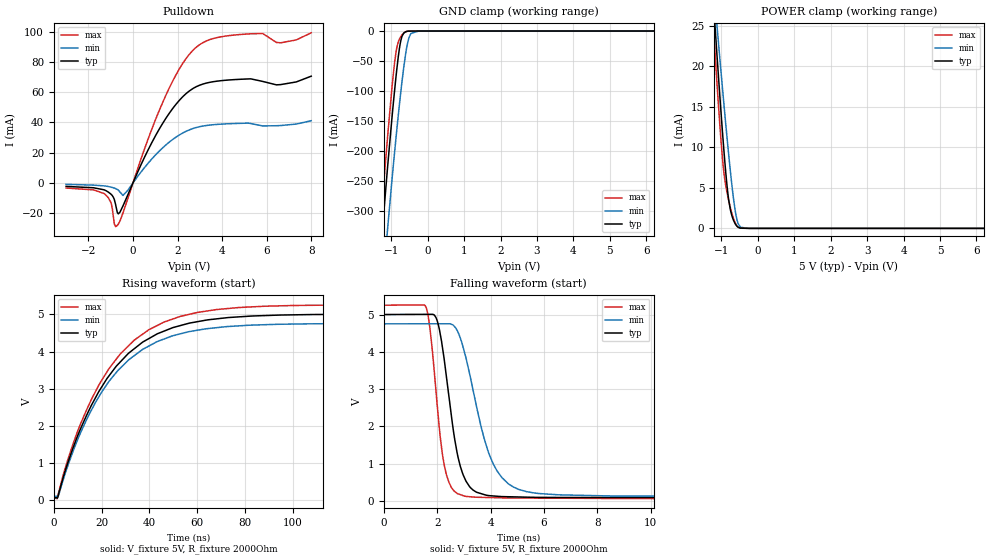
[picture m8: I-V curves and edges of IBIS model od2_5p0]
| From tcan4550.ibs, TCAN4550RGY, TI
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|   od2_5p0 Model
[Model]   od2_5p0
Model_type   Open_drain
Polarity   Non-Inverting
Vmeas = 2.5
Vref = 5
Cref = 2pF
Rref = 2000
|   typ   min   max
C_comp   6.451pF   6.048pF   6.601pF
|  Where Nom  PVT is Nominal Process, 5V,   27C
|   Fast PVT is Strong Process,  5.25, -40C
|   Slow PVT is Weak Process,   4.75V, 150C
[Voltage Range]   5   4.75   5.25
|Junction Temperature
[Temperature Range]   27   150   -40
[Pullup Reference]   5   4.75   5.25
[Pulldown Reference]   0   0   0
[Power Clamp Reference]   5   4.75   5.25
[GND Clamp Reference]   0   0   0
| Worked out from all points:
|   slope of the pulldown table from 0 to 0.75 V, typ, clamps not added: 31.4 ohm
|   GND clamp passes 1 mA (typ) near -0.60 V on its own axis
|   POWER clamp passes 1 mA (typ) near -0.67 V on its own axis
|   falling waveform, V_fixture 5V, R_fixture 2000Ohm: 20-80 % time 602ps typ, 987ps min, 438ps max; typ from 5 V to 0.072 V
|   rising waveform, V_fixture 5V, R_fixture 2000Ohm: 20-80 % time 26.4ns typ, 25.8ns min, 26.3ns max; typ from 0.072 V to 5 V
[Pulldown]
|   Voltage   I(typ)   I(min)   I(max)
-3V       -2.248mA   -898uA     -3.336mA
-1.295V   -4.511mA   -1.914mA   -6.963mA
-987mV    -7.375mA   -2.744mA   -12.99mA
-767mV    -15.07mA   -3.769mA   -28.8mA
-580mV    -19.24mA   -6.009mA   -25.08mA
-448mV    -15.19mA   -8.232mA   -19.84mA
1.301V    38.61mA    22.78mA    52.14mA
2.72V     62.7mA     36.15mA    88.14mA
4.117V    67.88mA    39.05mA    97.06mA
5.822V    67.15mA    37.74mA    98.84mA
6.636V    65.08mA    37.99mA    92.71mA
8V        70.63mA    41.17mA    99.3mA
[GND Clamp]
|   Voltage   I(typ)   I(min)   I(max)
-3V       -1.787A    -1.824A    -1.779A
-1.537V   -564.5mA   -655.4mA   -521.4mA
-1.262V   -347mA     -447.2mA   -298.1mA
-1.229V   -321.9mA   -422.9mA   -272.5mA
-1.097V   -225mA     -328.3mA   -174.4mA
-954mV    -128.1mA   -231.7mA   -78.72mA
-866mV    -74.34mA   -176.2mA   -33.94mA
-734mV    -15.3mA    -99.82mA   -9.032mA
-602mV    -1.078mA   -37.05mA   -1.282mA
-459mV    -34.02uA   -3.944mA   -29.01uA
-239mV    0A         -15.58uA   0A
8V        0A         0A         0A
[POWER Clamp]
|   Voltage   I(typ)   I(min)   I(max)
-3V       155.6mA    128.7mA    164.6mA
-1.218V   27.88mA    30.1mA     24.84mA
-1.163V   24.19mA    27.21mA    20.89mA
-1.108V   20.57mA    24.34mA    17.06mA
-1.009V   14.27mA    19.27mA    10.74mA
-943mV    10.33mA    15.96mA    7.398mA
-811mV    3.932mA    9.64mA     3.677mA
-756mV    2.375mA    7.19mA     2.613mA
-668mV    1.014mA    3.702mA    1.225mA
-536mV    132.5uA    547.2uA    135.2uA
-239mV    0A         472.1nA    0A
8V        0A         0A         0A
[Ramp]
R_load = 2000
|   typ   min   max
dV/dt_r   2.95704/2.63812e-08   2.78269/2.58481e-08   3.11551/2.634e-08
dV/dt_f   2.95704/6.00476e-10   2.78269/9.85701e-10   3.11551/4.37201e-10
[Falling Waveform]
V_fixture = 5V
V_fixture_min = 4.75V
V_fixture_max = 5.25V
R_fixture = 2000Ohm
C_fixture = 0F
|   Time   V(typ)   V(min)   V(max)
0s        5V         4.75V      5.25V
1.573ns   5.005V     4.751V     5.205V
1.957ns   4.911V     4.751V     2.897V
2.214ns   4.018V     4.752V     1.15V
2.688ns   1.508V     4.644V     229.4mV
3.233ns   362mV      3.341V     109.2mV
3.89ns    144.9mV    1.36V      89.51mV
4.443ns   113.4mV    610mV      79.94mV
23.1ns    71.73mV    112.1mV    57.53mV
500ns     71.6mV     112.2mV    57.49mV
[Rising Waveform]
V_fixture = 5V
V_fixture_min = 4.75V
V_fixture_max = 5.25V
R_fixture = 2000Ohm
C_fixture = 0F
|   Time   V(typ)   V(min)   V(max)
0s        71.6mV     112.2mV    57.49mV
1.964ns   159.9mV    132.7mV    193.5mV
7.423ns   1.298V     1.209V     1.397V
14.32ns   2.367V     2.247V     2.517V
20.17ns   3.059V     2.923V     3.238V
27.71ns   3.711V     3.545V     3.925V
39.84ns   4.348V     4.148V     4.587V
60.06ns   4.8V       4.57V      5.049V
116.4ns   4.996V     4.747V     5.247V
500ns     5V         4.75V      5.25V
